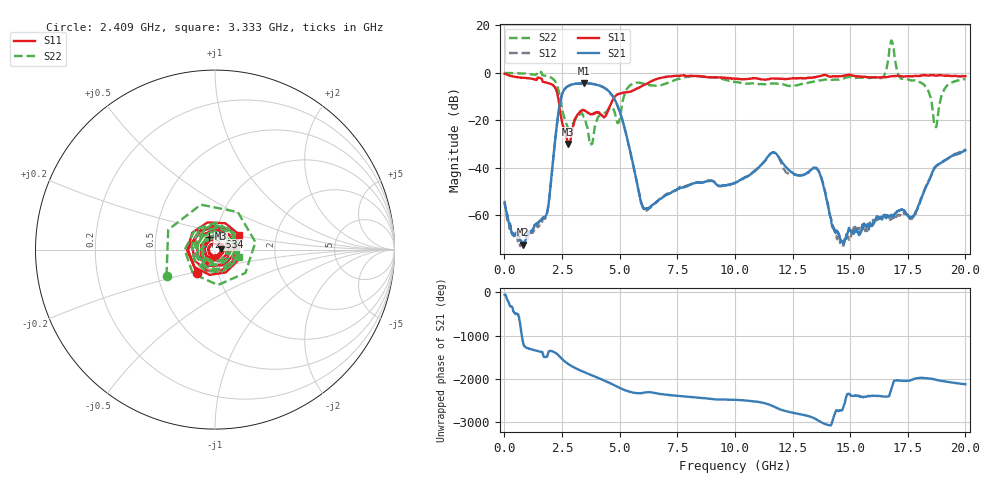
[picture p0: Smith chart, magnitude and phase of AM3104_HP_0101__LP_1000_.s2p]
!Created with skrf (http://scikit-rf.org).
# Hz S RI R 50.0
!freq ReS11 ImS11 ReS21 ImS21 ReS12 ImS12 ReS22 ImS22
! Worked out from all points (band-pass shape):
!   1601 points, 10 MHz to 20 GHz, reference 50 ohm
!   highest |S21| = -4.35 dB at 3.446 GHz (marker M1); lowest = -72.3 dB at 822.1 MHz (marker M2)
!   |S21| within 3 dB of the highest: 2.579 GHz to 4.493 GHz (1.914 GHz wide, 54.1 % of centre)
!   lowest |S11| = -29.9 dB at 2.771 GHz (marker M3), VSWR 1.07, Z = 53.3 + j0.613 ohm
!   |S11| at or under -10 dB: 2.325 GHz to 4.79 GHz (2.465 GHz wide, 69.3 % of centre)
!   |S22| runs from -30.3 to 13.7 dB; largest |S21 - S12| = 0.044
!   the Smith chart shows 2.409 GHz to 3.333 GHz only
!   S11 on the Smith chart (normalised r, x): 2.409 GHz: 0.79, -0.21; 2.534 GHz: 0.92, +0.13; 3.333 GHz: 1.29, +0.22
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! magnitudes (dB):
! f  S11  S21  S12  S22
! 10 MHz  -0.4  -54.7  -53.8  0.0
! 822.1 MHz  -2.0  -72.3  -71.4  -0.2
! 1.834 GHz  -4.1  -59.4  -59.7  -1.3
! 2.409 GHz  -15.5  -12.8  -12.8  -10.3
! 2.534 GHz  -22.1  -8.2  -8.3  -16.5
! 2.771 GHz  -29.9  -5.5  -5.5  -23.3
! 3.333 GHz  -16.0  -4.4  -4.5  -17.0
! 3.346 GHz  -15.9  -4.4  -4.5  -16.9
! 3.446 GHz  -15.7  -4.4  -4.4  -18.6
! 3.771 GHz  -17.4  -4.6  -4.6  -29.8
! 4.708 GHz  -11.3  -9.9  -10.0  -15.0
! 6.007 GHz  -5.3  -56.5  -56.7  -4.5
! 6.682 GHz  -2.3  -53.7  -53.6  -5.3
! 10.01 GHz  -2.5  -46.4  -46.3  -3.9
! 11.64 GHz  -2.4  -33.5  -33.5  -4.4
! 13.34 GHz  -2.1  -40.5  -40.6  -3.8
! 14.63 GHz  -1.3  -70.9  -72.1  -2.6
! 16.68 GHz  -1.6  -60.9  -60.8  7.3
! 17.73 GHz  -1.4  -60.5  -60.5  -3.2
! 18.7 GHz  -1.2  -39.4  -39.6  -22.6
! 19.14 GHz  -1.1  -36.7  -36.5  -6.2
! 20 GHz  -1.4  -32.6  -32.3  -2.6
